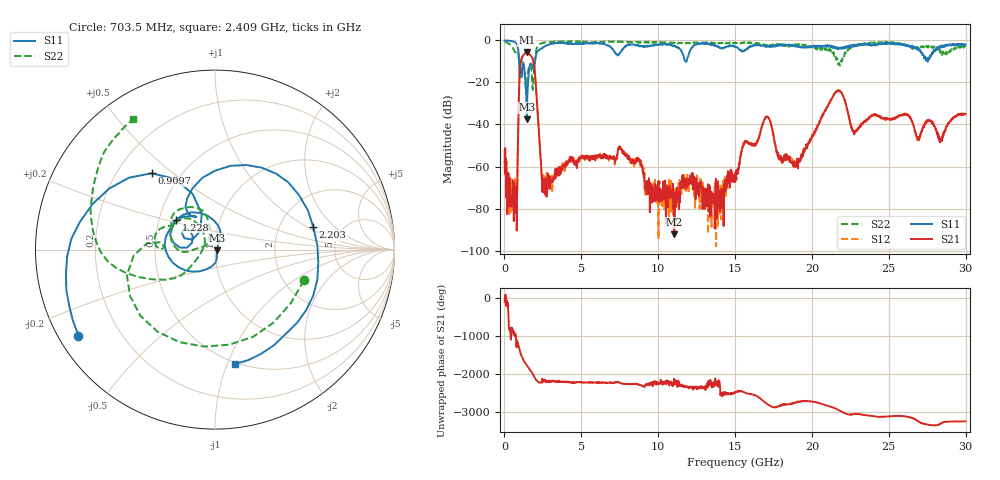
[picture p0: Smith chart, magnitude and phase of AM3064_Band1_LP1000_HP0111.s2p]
# Hz S DB R 50.0
!freq dBS11 angS11 dBS21 angS21 dBS12 angS12 dBS22 angS22
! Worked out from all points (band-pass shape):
!   1600 points, 10 MHz to 29.98 GHz, reference 50 ohm
!   highest |S21| = -5.72 dB at 1.453 GHz (marker M1); lowest = -92.3 dB at 11.05 GHz (marker M2)
!   |S21| within 3 dB of the highest: 1.111 GHz to 1.83 GHz (718.4 MHz wide, 48.9 % of centre)
!   lowest |S11| = -37.5 dB at 1.453 GHz (marker M3), VSWR 1.03, Z = 51.3 - j0.347 ohm
!   |S11| at or under -10 dB: 949.5 MHz to 1.993 GHz (1.044 GHz wide, 70.9 % of centre); 11.78191 GHz to 11.83991 GHz (58 MHz wide, 0.491 % of centre); 27.52508 GHz to 27.5452 GHz (20.12 MHz wide, 0.0731 % of centre)
!   |S22| runs from -25.2 to -0.4 dB; largest |S21 - S12| = 0.0064
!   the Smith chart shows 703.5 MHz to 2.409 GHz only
!   S11 on the Smith chart (normalised r, x): 703.5 MHz: 0.06, -0.29; 909.7 MHz: 0.35, +0.42; 1.228 GHz: 0.61, +0.22; 2.203 GHz: 3.11, +1.14; 2.409 GHz: 0.49, -1.07
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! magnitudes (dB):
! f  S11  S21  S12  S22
! 10 MHz  0.0  -52.9  -57.2  -0.4
! 703.5 MHz  -0.9  -72.3  -82.9  -5.6
! 909.7 MHz  -5.1  -36.2  -36.1  -6.9
! 1.06 GHz  -13.7  -10.6  -10.6  -9.6
! 1.228 GHz  -11.2  -7.0  -7.0  -10.8
! 1.453 GHz  -37.5  -5.7  -5.7  -21.8
! 1.884 GHz  -13.5  -10.1  -10.2  -18.3
! 2.203 GHz  -5.0  -39.3  -39.0  -2.3
! 2.409 GHz  -3.8  -61.9  -62.9  -1.3
! 5.015 GHz  -1.4  -55.7  -55.0  -0.7
! 7.526 GHz  -5.7  -51.5  -50.7  -0.7
! 10 GHz  -2.0  -71.3  -77.0  -0.9
! 11.05 GHz  -2.4  -92.3  -72.1  -1.2
! 15 GHz  -3.0  -67.4  -62.7  -1.4
! 17.03 GHz  -3.1  -36.3  -36.3  -2.4
! 17.99 GHz  -2.4  -55.4  -57.2  -2.3
! 19.99 GHz  -3.2  -46.0  -46.2  -3.2
! 21.68 GHz  -4.3  -23.8  -23.9  -9.8
! 22.75 GHz  -3.0  -44.7  -43.1  -2.0
! 25 GHz  -1.1  -37.4  -37.4  -1.1
! 28.35 GHz  -3.6  -47.7  -47.5  -5.9
! 29.98 GHz  -1.9  -34.9  -35.0  -3.1
